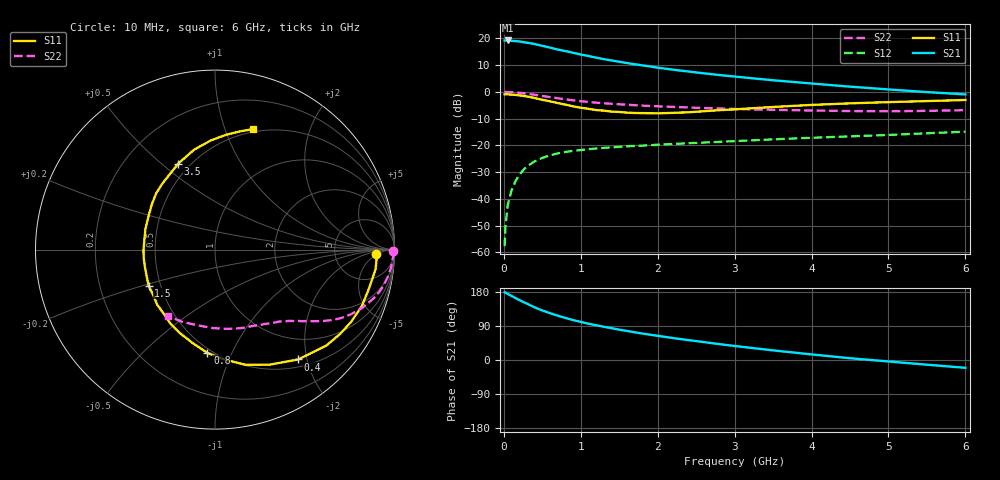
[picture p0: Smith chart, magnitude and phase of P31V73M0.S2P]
! SIEMENS Small Signal Semiconductors
! BFP181
! Si NPN RF Bipolar Junction Transistor in SOT143
! VCE = 1.75 V  IC = 3 mA
! Common Emitter S-Parameters:  March  1996
# GHz  S  MA  R  50
!  f  S11  S21  S12  S22
! GHz  MAG  ANG  MAG  ANG  MAG  ANG  MAG  ANG
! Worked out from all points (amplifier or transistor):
!   36 points, 10 MHz to 6 GHz, reference 50 ohm
!   highest |S21| = 19.2 dB at 50 MHz (marker M1)
!   |S21| within 3 dB of that: start of sweep to 645.2 MHz
!   unconditionally stable (mu >= 1): 2.001 GHz to end of sweep
!   at 250 MHz: K = 0.16, MSG = 24.0 dB, |S12| = -29.3 dB
!   at 1.4 GHz: K = 0.78, MSG = 16.2 dB, |S12| = -20.8 dB
!   at 6 GHz: K = 1.10, MAG = 5.1 dB, |S12| = -14.9 dB
!   S11 on the Smith chart (normalised r, x): 10 MHz: 17, -5; 400 MHz: 0.62, -1.85; 800 MHz: 0.47, -0.81; 1.5 GHz: 0.43, -0.21; 3.5 GHz: 0.43, +0.57; 6 GHz: 0.47, +1.25
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0.01  0.8993 -1.7  9.097 179.0  0.0013 89.6  0.9945 -0.6
0.02  0.9022 -3.0  9.06 178.3  0.0029 87.5  0.9958 -1.2
0.05  0.9012 -6.9  9.14 174.5  0.0076 88.5  0.9911 -3.1
0.1  0.885 -14.1  8.984 169.1  0.0143 81.9  0.985 -6.1
0.2  0.8593 -27.8  8.783 158.3  0.0279 73.9  0.9599 -12.1
0.25  0.8405 -34.0  8.502 153.3  0.0341 70.8  0.9428 -14.8
0.4  0.7675 -52.9  7.842 139.0  0.0501 61.1  0.8814 -21.7
0.5  0.7098 -64.6  7.248 130.6  0.0582 55.3  0.8367 -25.6
0.6  0.6651 -74.9  6.726 123.6  0.0653 51.0  0.7964 -28.7
0.7  0.6168 -84.7  6.174 117.0  0.0705 47.4  0.759 -31.2
0.8  0.5769 -94.2  5.783 111.0  0.0751 44.1  0.7257 -33.2
0.9  0.5353 -103.5  5.382 105.4  0.0789 41.4  0.6948 -35.0
1.1  0.4813 -121.0  4.682 95.7  0.0846 37.5  0.6468 -38.0
1.3  0.4452 -136.3  4.09 87.7  0.0896 34.3  0.6121 -40.5
1.5  0.4207 -151.6  3.656 80.0  0.0936 32.4  0.5852 -42.8
1.8  0.4 -172.9  3.124 69.8  0.0987 30.5  0.5525 -46.1
2.2  0.4044 163.6  2.596 57.9  0.106 28.2  0.5232 -51.1
2.8  0.454 136.1  2.062 41.9  0.116 25.9  0.4884 -59.5
3.5  0.5213 113.1  1.646 25.4  0.1293 23.3  0.4618 -71.2
4.5  0.6091 92.1  1.251 4.7  0.147 18.9  0.4375 -91.7
5.5  0.6721 78.3  0.99 -12.4  0.168 14.8  0.4411 -113.9
6  0.7038 72.5  0.895 -20.6  0.1798 12.1  0.4538 -125.1
